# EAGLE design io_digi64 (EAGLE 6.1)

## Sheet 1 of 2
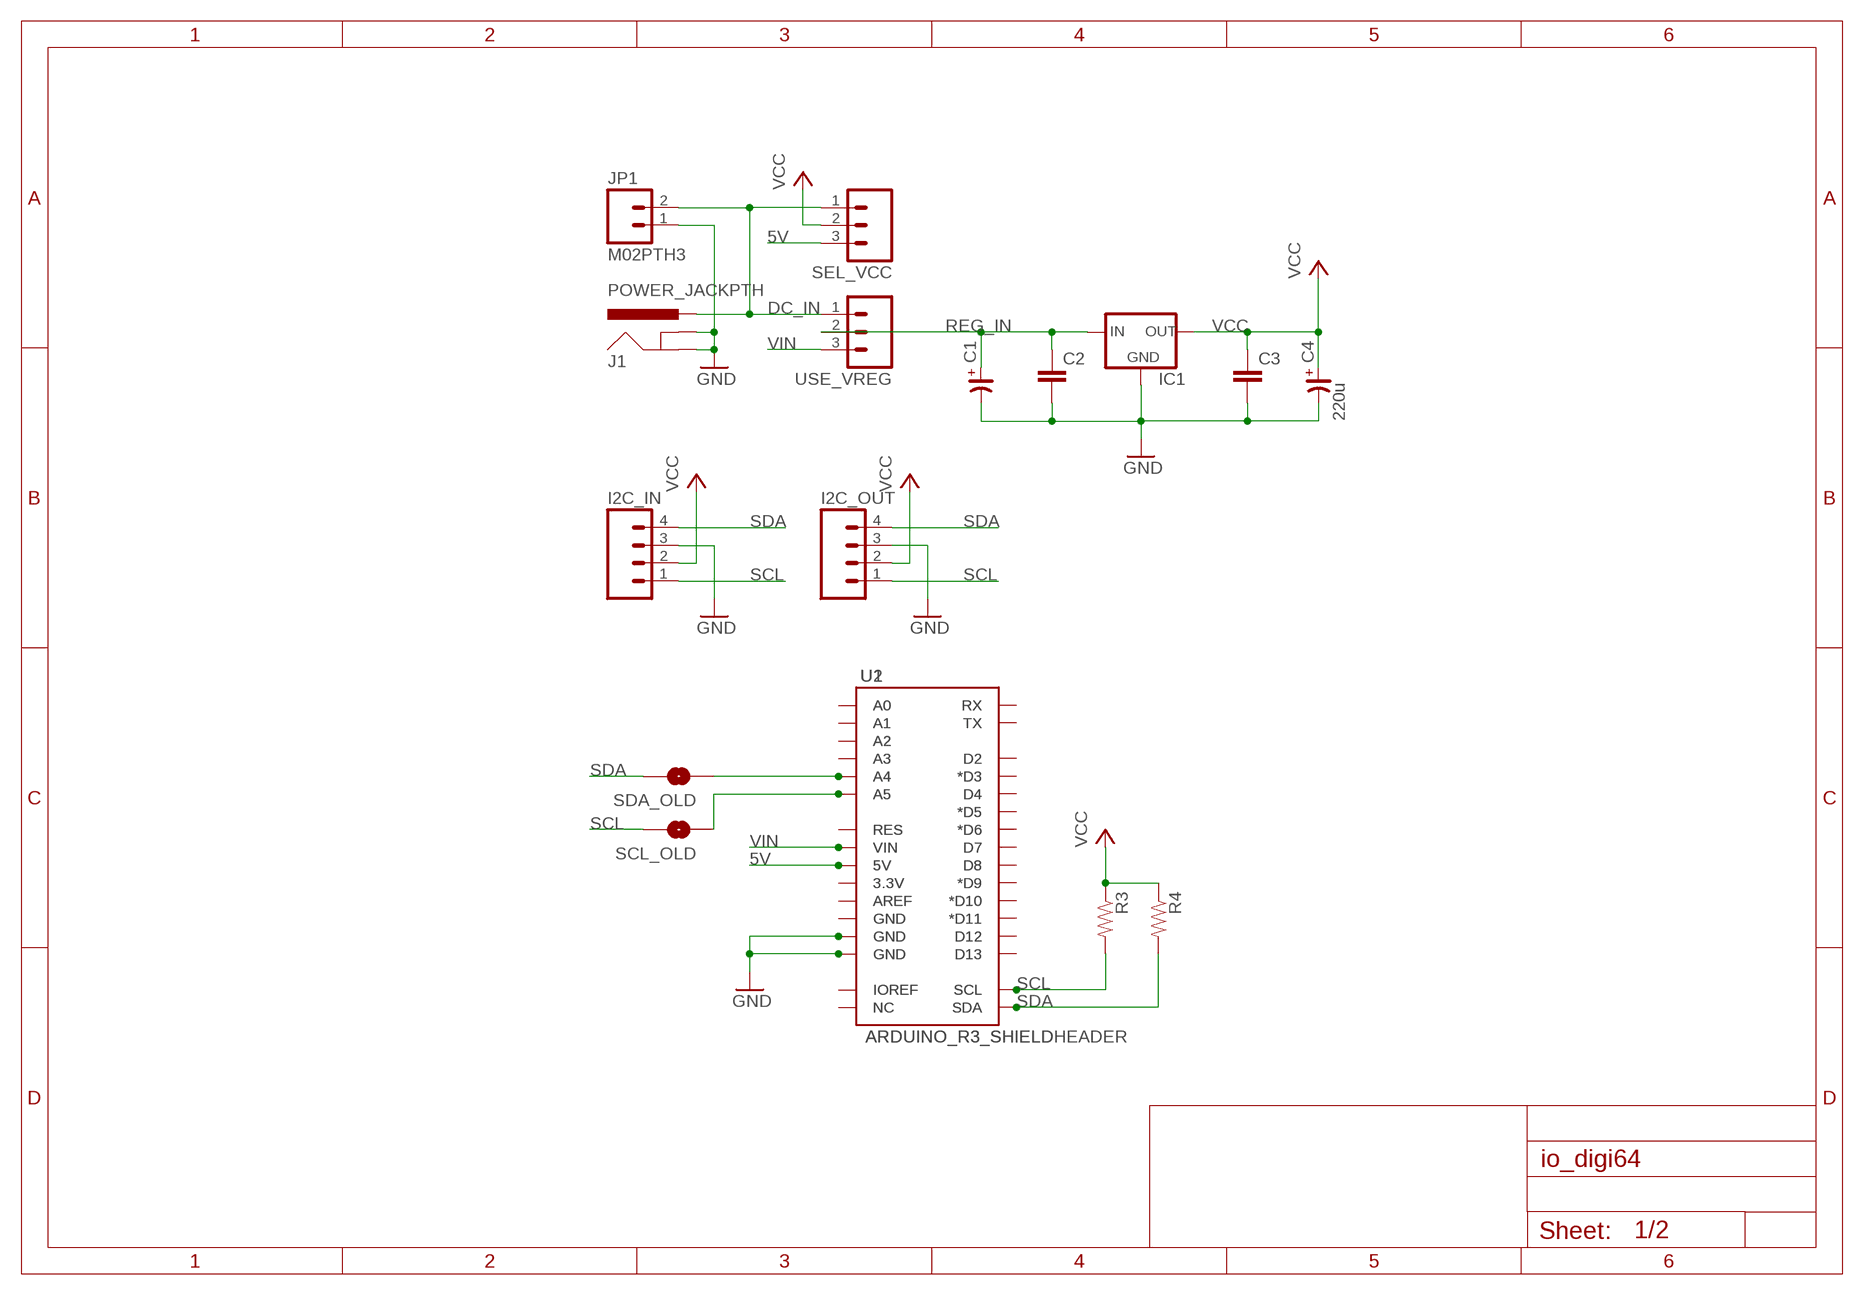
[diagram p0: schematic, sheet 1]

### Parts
C1  CP_E-025X065  [CE-025X065]
C2  CAPPTH1  [CAP-PTH-5MM]
C3  CAPPTH1  [CAP-PTH-5MM]
C4  220u  CP_E-035X080  [CE-035X080]
I2C_IN  M04PTH  [1X04]
I2C_OUT  M04PTH  [1X04]
IC1  V_REG_78XXSINK  [TO220-IGO]
J1  POWER_JACKPTH  [POWER_JACK_PTH]
JP1  M02PTH3  [1X02_LONGPADS]
R3  RESISTORPTH-1/6W  [1/6W-RES]
R4  RESISTORPTH-1/6W  [1/6W-RES]
SCL_OLD  SOLDERJUMPERNO  [SJ_2S-NO]
SDA_OLD  SOLDERJUMPERNO  [SJ_2S-NO]
SEL_VCC  M03PTH  [1X03]
U1  ARDUINO_R3_SHIELD  [ARDUINOR3_NOHOLE_NOLABELS]
U2  ARDUINO_R3_SHIELDHEADER  [ARDUINOR3_NODOC]
USE_VREG  M03PTH  [1X03]

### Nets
5V: SEL_VCC.3 U1.5V U2.5V
DC_IN: J1.PWR JP1.2 SEL_VCC.1 USE_VREG.1
GND [power]: C1.- C2.2 C3.2 C4.- I2C_IN.3 I2C_OUT.3 IC1.GND J1.GND J1.GNDBREAK JP1.1 U1.GND@0(GND) U1.GND@1(GND) U2.GND@0(GND) U2.GND@1(GND) ; also sheet 2
N$57: SDA_OLD.1 U1.A4 U2.A4
N$58: SCL_OLD.1 U1.A5 U2.A5
N$59: U1.NC U2.NC
N$60: U1.RX U2.RX
N$61: U1.TX U2.TX
N$62: U1.D2 U2.D2
N$63: U1.D3(*D3) U2.D3(*D3)
N$64: U1.D4 U2.D4
N$65: U1.D5(*D5) U2.D5(*D5)
N$66: U1.D6(*D6) U2.D6(*D6)
N$67: U1.D7 U2.D7
N$68: U1.D8 U2.D8
N$69: U1.D9(*D9) U2.D9(*D9)
N$70: U1.D10(*D10) U2.D10(*D10)
N$71: U1.D11(*D11) U2.D11(*D11)
N$72: U1.D12 U2.D12
N$73: U1.D13 U2.D13
N$74: U1.A0 U2.A0
N$75: U1.A1 U2.A1
N$76: U1.A2 U2.A2
N$77: U1.A3 U2.A3
N$79: U1.RES U2.RES
N$81: U1.AREF U2.AREF
N$82: U1.GND@2(GND) U2.GND@2(GND)
N$83: U1.3.3V U2.3.3V
N$84: U1.IOREF U2.IOREF
REG_IN: C1.+ C2.1 IC1.IN USE_VREG.2
SCL: I2C_IN.1 I2C_OUT.1 R3.2 SCL_OLD.2 U1.SCL U2.SCL ; also sheet 2
SDA: I2C_IN.4 I2C_OUT.4 R4.2 SDA_OLD.2 U1.SDA U2.SDA ; also sheet 2
VCC [power]: C3.1 C4.+ I2C_IN.2 I2C_OUT.2 IC1.OUT R3.1 R4.1 SEL_VCC.2 ; also sheet 2
VIN [power]: U1.VIN U2.VIN USE_VREG.3

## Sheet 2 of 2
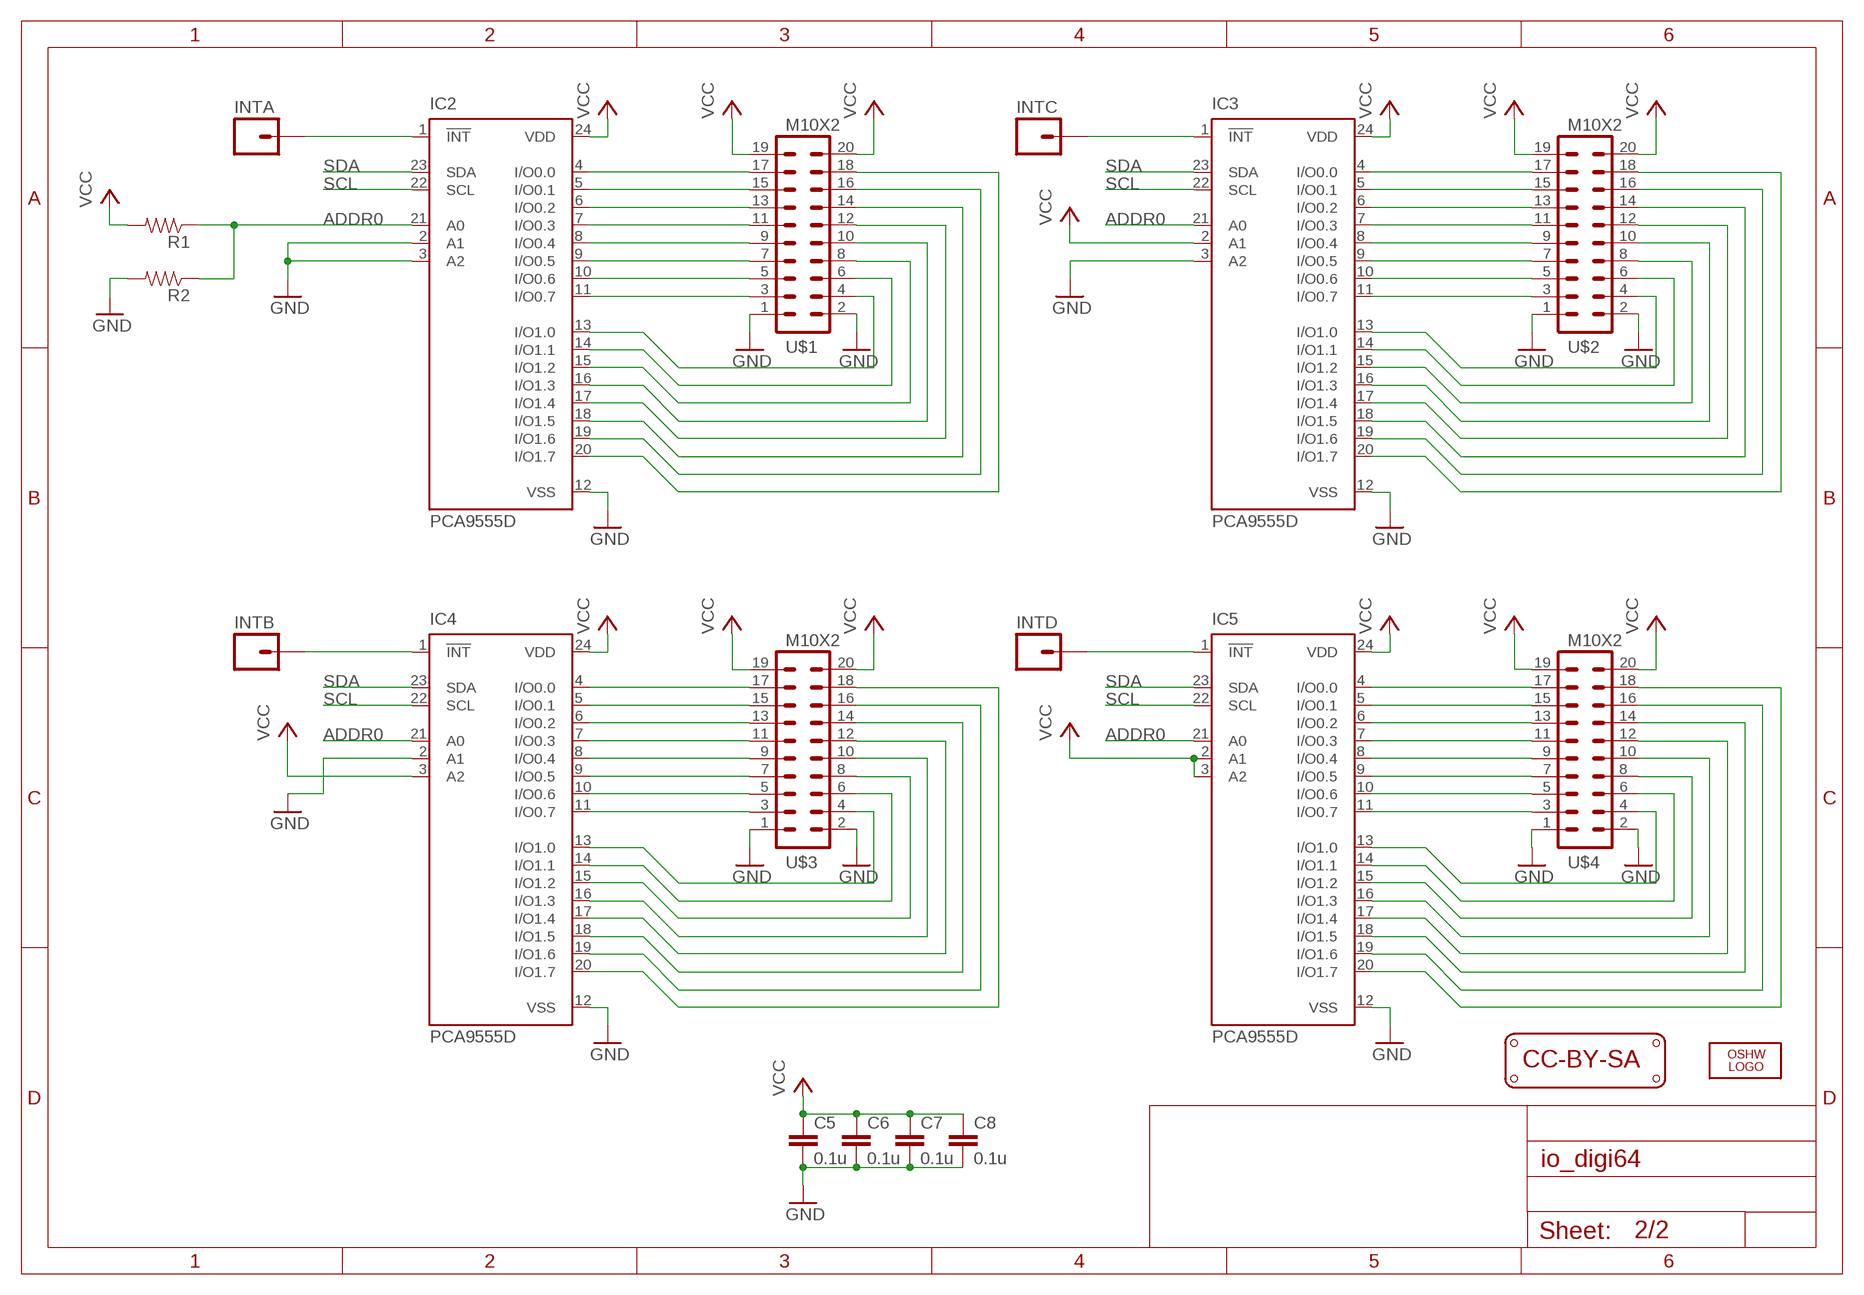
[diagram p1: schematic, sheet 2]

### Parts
C5  0.1u  CAP0805  [0805]
C6  0.1u  CAP0805  [0805]
C7  0.1u  CAP0805  [0805]
C8  0.1u  CAP0805  [0805]
IC2  PCA9555D  [SO24]
IC3  PCA9555D  [SO24]
IC4  PCA9555D  [SO24]
IC5  PCA9555D  [SO24]
INTA  M01PTH  [1X01]
INTB  M01PTH  [1X01]
INTC  M01PTH  [1X01]
INTD  M01PTH  [1X01]
LOGO1  LOGO_CC-BY-SA  [CC-BY-SA]
LOGO2  OSHW_LOGO_FILLX0200-NT  [OSHW_FILLX200_NOTEXT]
R1  RESISTORPTH-1/6W  [1/6W-RES]
R2  RESISTORPTH-1/6W  [1/6W-RES]
U$1  M10X2  [2X10]
U$2  M10X2  [2X10]
U$3  M10X2  [2X10]
U$4  M10X2  [2X10]

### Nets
ADDR0: IC2.21(A0) IC3.21(A0) IC4.21(A0) IC5.21(A0) R1.1 R2.1
GND [power]: C5.2 C6.2 C7.2 C8.2 IC2.2(A1) IC2.3(A2) IC2.12(VSS) IC3.3(A2) IC3.12(VSS) IC4.2(A1) IC4.12(VSS) IC5.12(VSS) R2.2 U$1.1 U$1.2 U$2.1 U$2.2 U$3.1 U$3.2 U$4.1 U$4.2 ; also sheet 1
N$1: IC4.13(I/O1.0) U$3.4
N$2: IC4.14(I/O1.1) U$3.6
N$3: IC4.15(I/O1.2) U$3.8
N$4: IC4.16(I/O1.3) U$3.10
N$5: IC4.17(I/O1.4) U$3.12
N$6: IC4.18(I/O1.5) U$3.14
N$7: IC4.19(I/O1.6) U$3.16
N$8: IC4.20(I/O1.7) U$3.18
N$9: IC3.11(I/O0.7) U$2.3
N$10: IC3.10(I/O0.6) U$2.5
N$11: IC3.9(I/O0.5) U$2.7
N$12: IC3.8(I/O0.4) U$2.9
N$13: IC3.7(I/O0.3) U$2.11
N$14: IC3.6(I/O0.2) U$2.13
N$15: IC3.5(I/O0.1) U$2.15
N$16: IC3.4(I/O0.0) U$2.17
N$17: IC3.13(I/O1.0) U$2.4
N$18: IC3.14(I/O1.1) U$2.6
N$19: IC3.15(I/O1.2) U$2.8
N$20: IC3.16(I/O1.3) U$2.10
N$21: IC3.17(I/O1.4) U$2.12
N$22: IC3.18(I/O1.5) U$2.14
N$23: IC3.19(I/O1.6) U$2.16
N$24: IC3.20(I/O1.7) U$2.18
N$25: IC5.11(I/O0.7) U$4.3
N$26: IC5.10(I/O0.6) U$4.5
N$27: IC5.9(I/O0.5) U$4.7
N$28: IC5.8(I/O0.4) U$4.9
N$29: IC5.7(I/O0.3) U$4.11
N$30: IC5.6(I/O0.2) U$4.13
N$31: IC5.5(I/O0.1) U$4.15
N$32: IC5.4(I/O0.0) U$4.17
N$33: IC5.13(I/O1.0) U$4.4
N$34: IC5.14(I/O1.1) U$4.6
N$35: IC5.15(I/O1.2) U$4.8
N$36: IC5.16(I/O1.3) U$4.10
N$37: IC5.17(I/O1.4) U$4.12
N$38: IC5.18(I/O1.5) U$4.14
N$39: IC5.19(I/O1.6) U$4.16
N$40: IC5.20(I/O1.7) U$4.18
N$41: IC2.11(I/O0.7) U$1.3
N$42: IC2.10(I/O0.6) U$1.5
N$43: IC2.9(I/O0.5) U$1.7
N$44: IC2.8(I/O0.4) U$1.9
N$45: IC2.7(I/O0.3) U$1.11
N$46: IC2.6(I/O0.2) U$1.13
N$47: IC2.5(I/O0.1) U$1.15
N$48: IC2.4(I/O0.0) U$1.17
N$49: IC2.13(I/O1.0) U$1.4
N$50: IC2.14(I/O1.1) U$1.6
N$51: IC2.15(I/O1.2) U$1.8
N$52: IC2.16(I/O1.3) U$1.10
N$53: IC2.17(I/O1.4) U$1.12
N$54: IC2.18(I/O1.5) U$1.14
N$55: IC2.19(I/O1.6) U$1.16
N$56: IC2.20(I/O1.7) U$1.18
N$80: IC2.1(!INT) INTA.1
N$85: IC4.1(!INT) INTB.1
N$86: IC3.1(!INT) INTC.1
N$87: IC5.1(!INT) INTD.1
N$113: IC4.11(I/O0.7) U$3.3
N$114: IC4.10(I/O0.6) U$3.5
N$115: IC4.9(I/O0.5) U$3.7
N$116: IC4.8(I/O0.4) U$3.9
N$117: IC4.7(I/O0.3) U$3.11
N$118: IC4.6(I/O0.2) U$3.13
N$119: IC4.5(I/O0.1) U$3.15
N$120: IC4.4(I/O0.0) U$3.17
SCL: IC2.22(SCL) IC3.22(SCL) IC4.22(SCL) IC5.22(SCL) ; also sheet 1
SDA: IC2.23(SDA) IC3.23(SDA) IC4.23(SDA) IC5.23(SDA) ; also sheet 1
VCC [power]: C5.1 C6.1 C7.1 C8.1 IC2.24(VDD) IC3.2(A1) IC3.24(VDD) IC4.3(A2) IC4.24(VDD) IC5.2(A1) IC5.3(A2) IC5.24(VDD) R1.2 U$1.19 U$1.20 U$2.19 U$2.20 U$3.19 U$3.20 U$4.19 U$4.20 ; also sheet 1

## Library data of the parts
C1 C4 = rc-master:CP_: POLARIZED CAP
C2 C3 C5-C8 = general:CAP: Capacitor
I2C_IN I2C_OUT = SparkFun-Connectors:M04: Header 4 Standard 4-pin 0.1" header. Use with straight break away headers (SKU : PRT-00116), right angle break away headers (PRT-00553), swiss pins (PRT-00743), machine pins (PRT-00117), and female headers (PRT-00115). Molex polarized connector foot print use with SKU : PRT-08231 with associated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
IC1 = SparkFun-PowerIC:V_REG_78XX: Voltage Regulator Standard 7805 5V regulator. IGO (Input Ground Output). Spark Fun Electronics SKU : COM-00107
IC2-IC5 = micro-philips:PCA9555: 16-bit I2C and SMBus I/O port with interrupt Source: PCA9555_5.pdf; MPN: PCA9555DW; OC_FARNELL: 1408295; OC_NEWARK: 63K6067
INTA INTB INTC INTD = SparkFun-Connectors:M01: Header 1
J1 = SparkFun-Connectors:POWER_JACK: Power Jack This is the standard 5.5mm barrel jack for power. The PTH is the most common, proven, reliable, footprint. The Slot footprint only works if the mill layer is transmitted to the PCB fab house so be warned. Spark Fun Electronics SKU : PRT-00119 SMT: CONN-08106 Mating wall wart : TOL-00298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
JP1 = SparkFun-Connectors:M02: Standard 2-pin 0.1" header. Use with
LOGO1 = dp_devices:LOGO_CC-BY-SA
LOGO2 = ohw-logo:OSHW_LOGO_FILL
R1-R4 = general:RESISTOR: Resistor
SCL_OLD SDA_OLD = SparkFun-Passives:SOLDERJUMPER: Solder Jumper
SEL_VCC USE_VREG = SparkFun-Connectors:M03: Header 3 Standard 3-pin 0.1" header. Use with straight break away headers (SKU : PRT-00116), right angle break away headers (PRT-00553), swiss pins (PRT-00743), machine pins (PRT-00117), and female headers (PRT-00115). Molex polarized connector foot print use with SKU : PRT-08232 with associated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
U1 = arduino_shield:ARDUINO_R3_SHIELD; U: ArduinoR3
U2 = arduino_shield:ARDUINO_R3_SHIELD
U$1-U$4 = SparkFun-Connectors:M10X2: This was SPECIALLY designed to be used with our Graphic LCD Backpack. Be sure you want to use this! It is not only staggered on each line of header holes, but IT IS ALSO offset of the center point of the top and bottom lines by 5 mil. This causes the headers to lock into place on the "standard"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

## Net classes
1 power: width 0.406 mm, clearance 0.203 mm

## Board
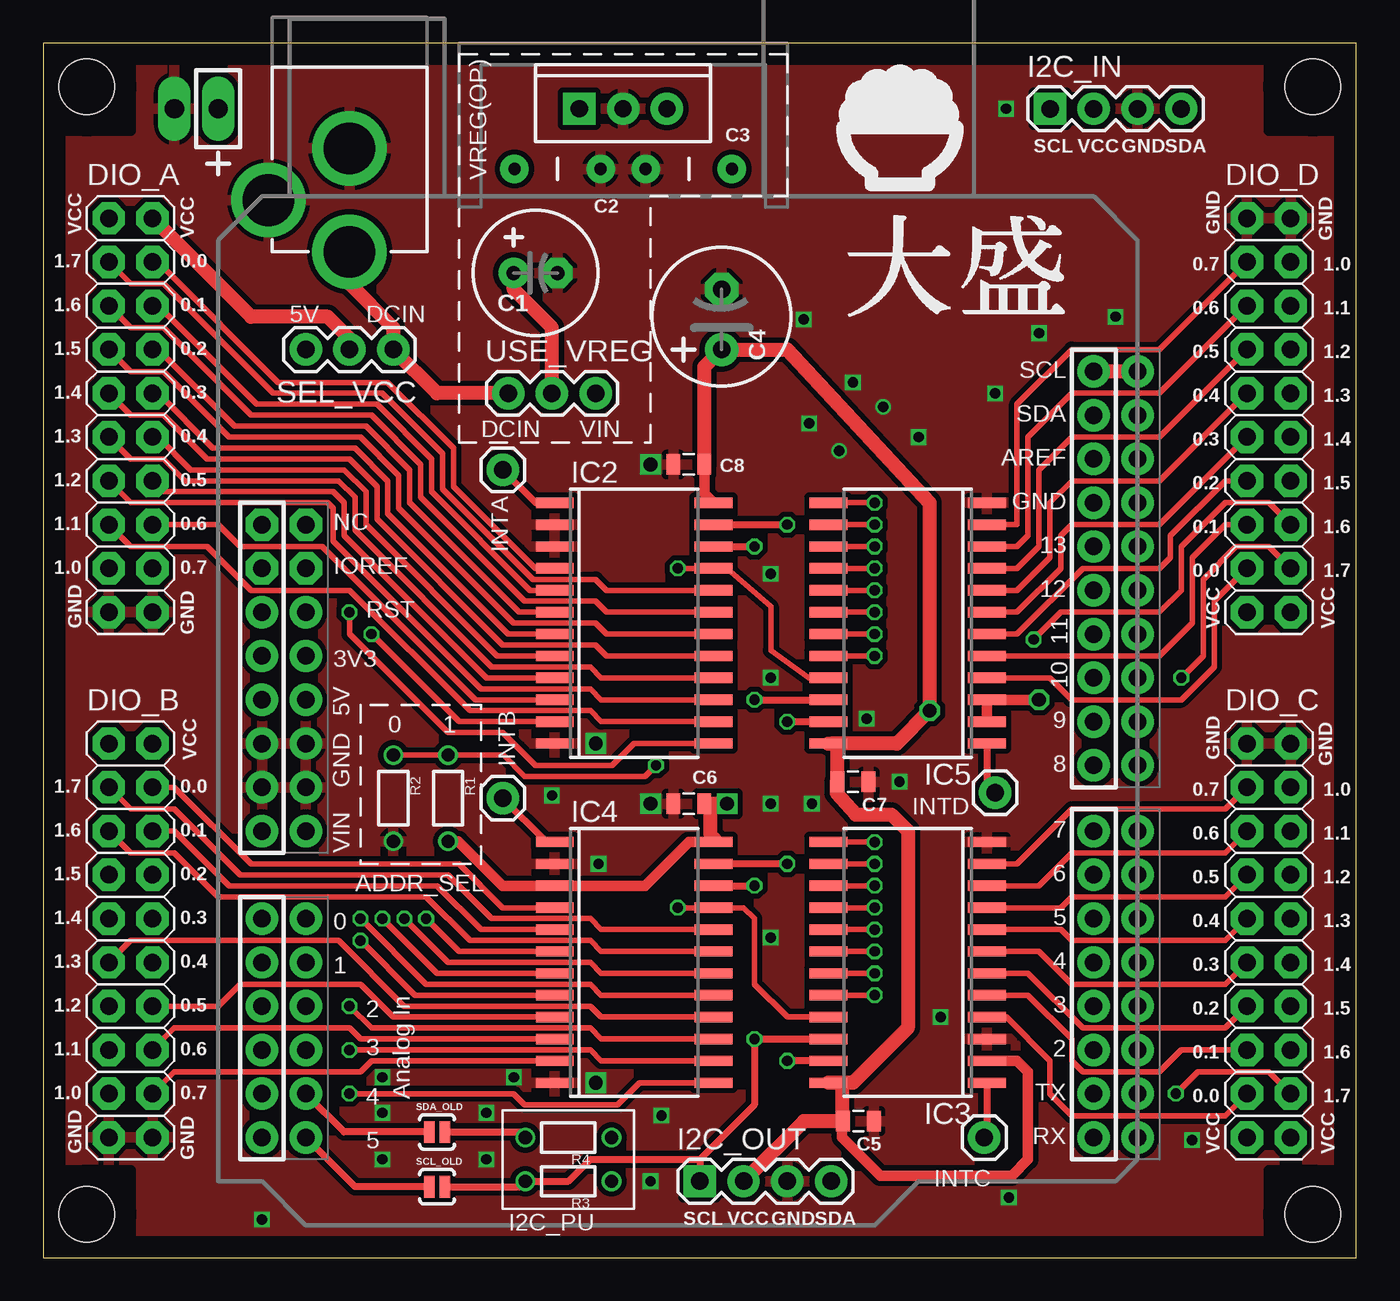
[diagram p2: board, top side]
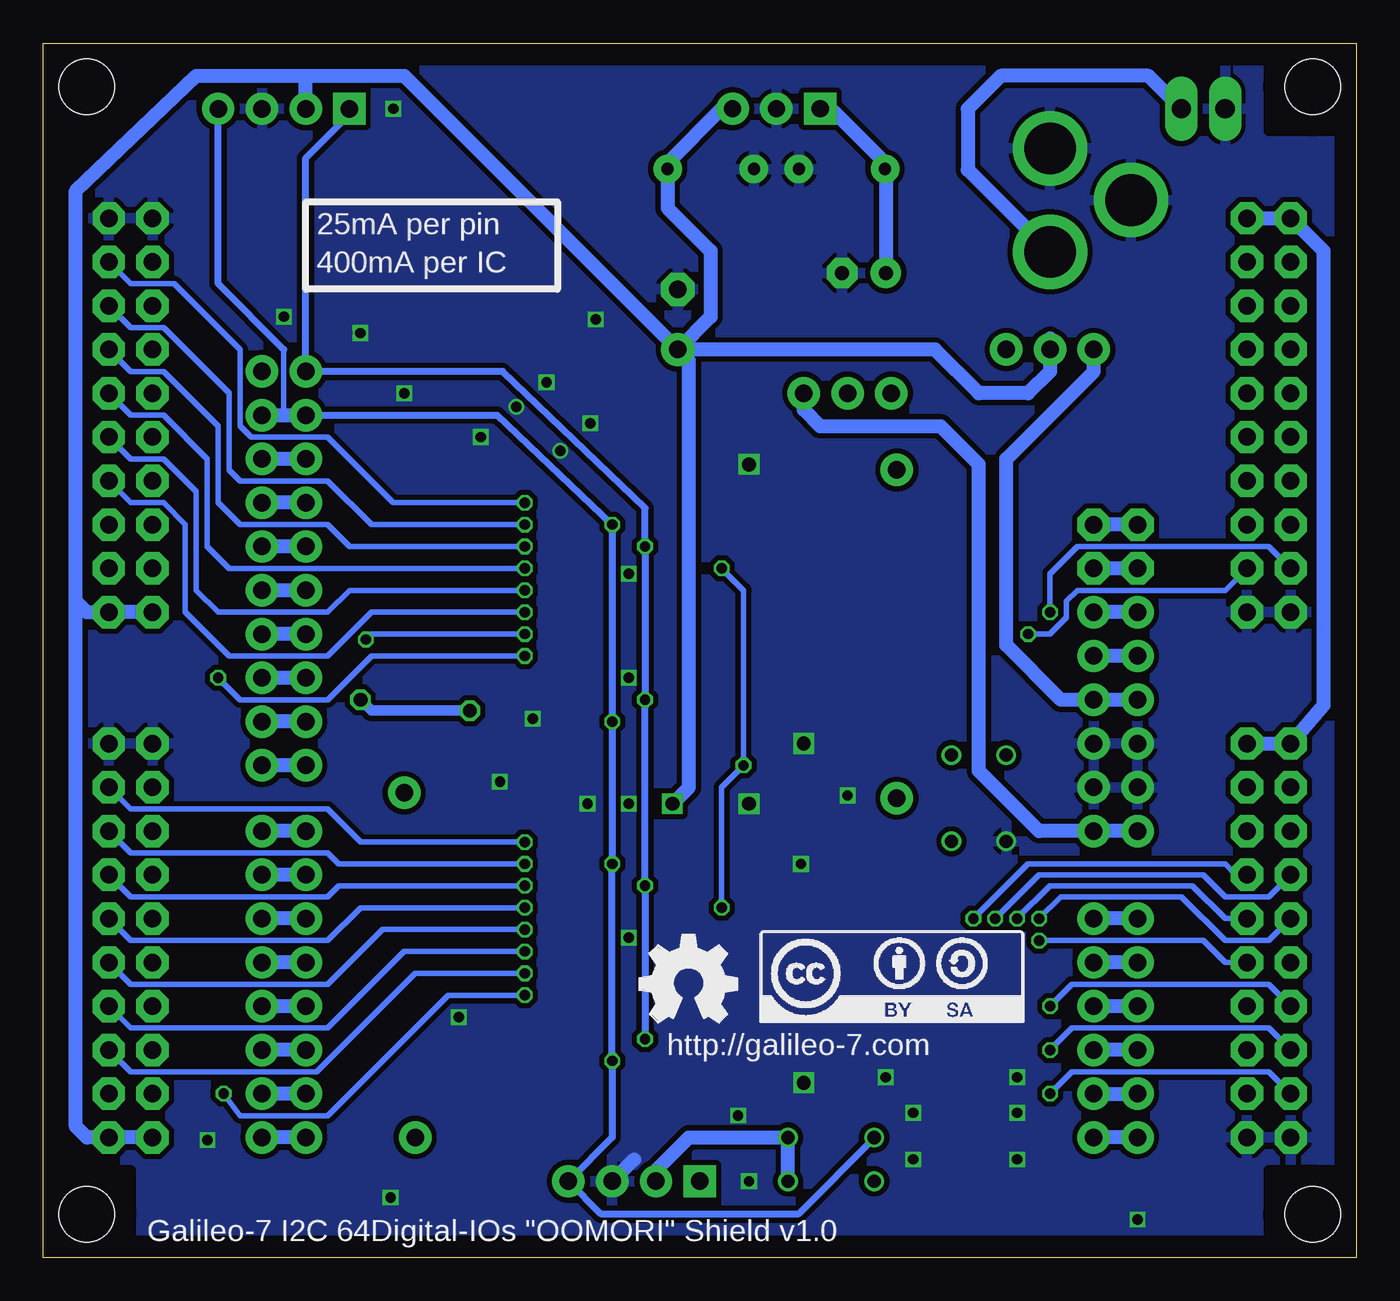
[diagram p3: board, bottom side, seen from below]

Size 76.2 x 70.48 mm. Coordinates in mm from the lower left corner, seen from the top.
Outline: 0,0 76.2,0 76.2,70.48 0,70.48 0,0
Copper layers (1*2*15*16): Top 0.035mm / dielectric 0.2mm / Route2 0.0175mm / dielectric 1.1mm / Route15 0.0175mm / dielectric 0.2mm / Bottom 0.035mm
Design rules: minimum track width 6mil, minimum drill 12mil, track to track 6mil, track to pad 6mil, pad to pad 6mil, via to via 6mil, smd to smd 0mil, copper to edge 50mil, drill to drill 10mil, minimum pad ring 6mil, minimum via ring 6mil, stop-mask expansion 2mil, vias tented up to drill 25mil, thermal gap 10mil
Holes 3.2 mm at 2.54,67.94 73.66,67.94 2.54,2.54 73.66,2.54
tRestrict: area 0,0 to 5.1,5.1; area 71.1,0 to 76.2,5.1; area 71.1,65.4 to 76.2,70.5; area 0,65.4 to 5.1,70.5
bRestrict: area 0,0 to 5.1,5.1; area 71.1,0 to 76.2,5.1; area 71.1,65.4 to 76.2,70.5; area 0,65.4 to 5.1,70.5

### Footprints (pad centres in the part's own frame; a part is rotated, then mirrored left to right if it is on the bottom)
CE-025X065 = drill 0.813 pad 1.778: + -1.27,0 | drill 0.813 pad 1.778 octagon: - 1.27,0
CAP-PTH-5MM = drill 0.7 pad 1.651: 1 -2.5,0; 2 2.5,0
CE-035X080 = drill 1.016 pad 1.93: + -1.905,0 | drill 1.016 pad 1.93 octagon: - 1.587,0
0805 = smd 0.8 x 1.2: 1 -0.9,0; 2 0.9,0
1X04 = drill 1.016 pad 1.88 square: 1 0,0 | drill 1.016 pad 1.88: 2 2.54,0; 3 5.08,0; 4 7.62,0
TO220-IGO = drill 1 pad 1.88: GND 0,0; OUT 2.54,0 | drill 1 pad 1.88 square: IN -2.54,0
SO24 = smd 0.6 x 2.2: 1 -6.985,-4.6; 2 -5.715,-4.6; 3 -4.445,-4.6; 4 -3.175,-4.6; 5 -1.905,-4.6; 6 -0.635,-4.6; 7 0.635,-4.6; 8 1.905,-4.6; 9 3.175,-4.6; 10 4.445,-4.6; 11 5.715,-4.6; 12 6.985,-4.6; 13 6.985,4.6; 14 5.715,4.6; 15 4.445,4.6; 16 3.175,4.6; 17 1.905,4.6; 18 0.635,4.6; 19 -0.635,4.6; 20 -1.905,4.6; 21 -3.175,4.6; 22 -4.445,4.6; 23 -5.715,4.6; 24 -6.985,4.6
1X01 = drill 1.016 pad 1.88: 1 0,0
POWER_JACK_PTH = drill 2.997 pad 4.318: GND 0,7.7; GNDBREAK 4.7,10.7; PWR 0,13.7
1X02_LONGPADS = drill 1.118 pad 1.88 long: 1 0,0; 2 2.54,0
1/6W-RES = drill 0.762: 1 -2.5,0; 2 2.5,0
SJ_2S-NO = smd 0.635 x 1.27: 1 -0.45,0; 2 0.45,0
1X03 = drill 1.016 pad 1.88: 1 0,0; 2 2.54,0; 3 5.08,0
ARDUINOR3_NOHOLE_NOLABELS = drill 1.016 pad 1.88: 3.3V 50.8,26.67; 5V 50.8,29.21; A0 50.8,41.91; A1 50.8,44.45; A2 50.8,46.99; A3 50.8,49.53; A4 50.8,52.07; A5 50.8,54.61; AREF 2.54,15.24; D2 2.54,49.53; D3 2.54,46.99; D4 2.54,44.45; D5 2.54,41.91; D6 2.54,39.37; D7 2.54,36.83; D8 2.54,33.02; D9 2.54,30.48; D10 2.54,27.94; D11 2.54,25.4; D12 2.54,22.86; D13 2.54,20.32; GND@0 50.8,31.75; GND@1 50.8,34.29; GND@2 2.54,17.78; RES 50.8,24.13; RX 2.54,54.61; SCL 2.54,10.16; SDA 2.54,12.7; TX 2.54,52.07; VIN 50.8,36.83 | drill 1.016 pad 1.88 octagon: IOREF 50.8,21.59; NC 50.8,19.05
ARDUINOR3_NODOC = drill 1.016 pad 1.88: 3.3V 50.8,26.67; 5V 50.8,29.21; A0 50.8,41.91; A1 50.8,44.45; A2 50.8,46.99; A3 50.8,49.53; A4 50.8,52.07; A5 50.8,54.61; AREF 2.54,15.24; D2 2.54,49.53; D3 2.54,46.99; D4 2.54,44.45; D5 2.54,41.91; D6 2.54,39.37; D7 2.54,36.83; D8 2.54,33.02; D9 2.54,30.48; D10 2.54,27.94; D11 2.54,25.4; D12 2.54,22.86; D13 2.54,20.32; GND@0 50.8,31.75; GND@1 50.8,34.29; GND@2 2.54,17.78; RES 50.8,24.13; RX 2.54,54.61; SCL 2.54,10.16; SDA 2.54,12.7; TX 2.54,52.07; VIN 50.8,36.83 | drill 1.016 pad 1.88 octagon: IOREF 50.8,21.59; NC 50.8,19.05
2X10 = drill 1.016 pad 1.88 octagon: 1 -11.43,-1.27; 2 -11.43,1.27; 3 -8.89,-1.27; 4 -8.89,1.27; 5 -6.35,-1.27; 6 -6.35,1.27; 7 -3.81,-1.27; 8 -3.81,1.27; 9 -1.27,-1.27; 10 -1.27,1.27; 11 1.27,-1.27; 12 1.27,1.27; 13 3.81,-1.27; 14 3.81,1.27; 15 6.35,-1.27; 16 6.35,1.27; 17 8.89,-1.27; 18 8.89,1.27; 19 11.43,-1.27; 20 11.43,1.27

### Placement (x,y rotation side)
C1  28.57,57.15 0 top
C2  29.84,63.18 0 top
C3  37.47,63.18 180 top
C4  39.37,54.61 90 top
C5  47.31,7.94 0 top
C6  37.47,26.35 180 top
C7  46.99,27.62 0 top
C8  37.47,46.04 180 top
I2C_IN  58.42,66.67 0 top
I2C_OUT  38.1,4.45 0 top
IC1  33.66,66.67 0 top
IC2  34.29,36.83 270 top
IC3  50.16,17.14 90 top
IC4  34.29,17.14 270 top
IC5  50.16,36.83 90 top
INTA  26.67,45.72 0 top
INTB  26.67,26.67 0 top
INTC  54.61,6.99 0 top
INTD  55.24,26.99 0 top
J1  17.78,72.07 180 top
JP1  7.62,66.67 0 top
LOGO1  34.61,13.65 0 bottom
LOGO2  41.59,13.65 0 bottom
R1  23.5,26.67 270 top
R2  20.32,26.67 270 top
R3  30.48,4.45 180 top
R4  30.48,6.99 180 top
SCL_OLD  22.86,4.13 0 top
SDA_OLD  22.86,7.3 0 top
SEL_VCC  20.32,52.7 180 top
U1  63.5,61.59 180 top
U2  66.04,61.59 180 top
U$1  5.08,48.9 90 top
U$2  71.12,18.41 270 top
U$3  5.08,18.41 90 top
U$4  71.12,48.9 270 top
U$5  [OMORI_LOGO]  46.04,61.91 0 top
U$6  [OMORI_LOGO2]  46.67,54.61 0 top
USE_VREG  26.99,50.16 0 top

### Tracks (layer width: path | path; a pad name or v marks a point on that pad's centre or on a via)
5V
  Bottom 0.813: SEL_VCC.3 15.24,51.44 20.32,46.35 20.32,35.56 17.14,32.38 U2.5V U1.5V
ADDR0  (via drill 0.6)
  Top 0.305: 45.72,33.66 IC5.21 44.45,33.66 42.23,35.24 42.23,37.78 39.69,40.01 IC2.21 v36.83,40.01 | IC3.21 43.18,13.97 41.27,15.88 41.27,19.68 40.64,20.32 IC4.21 v36.83,20.32 | R2.1 R1.1 26.71,29.17 27.94,27.94 34.92,27.94 v35.56,28.57
  Bottom 0.305: v36.83,40.01 35.56,38.73 v35.56,28.57 36.83,27.3 v36.83,20.32
DC_IN
  Top 0.813: USE_VREG.1 22.86,50.16 SEL_VCC.1 20.32,53.98 17.78,56.52 J1.PWR
  Bottom 0.813: JP1.2 12.06,68.58 20.64,68.58 22.54,66.67 22.54,63.13 J1.PWR
GND  (via drill 0.6, 0.8)
  Top 0.406: IC2.3 30.16,41.27
  Bottom 0.813: I2C_OUT.3 41.91,5.71
  other vias: 32.07,29.84 32.07,10.16 35.24,46.04 35.24,26.35 57.78,53.66 55.88,66.67 46.99,50.8 55.24,50.16 44.45,48.42 62.23,54.61 42.23,39.69 42.23,33.66 42.23,26.35 42.23,18.57 46.2,46.83 48.74,49.37 29.53,26.83 35.88,8.26 27.3,10.48 19.68,10.48 44.13,54.45 47.78,31.27 56.04,3.49 32.23,22.86 50.8,47.62 44.61,26.35 49.69,27.62 52.07,13.97 12.7,2.22 66.67,6.83 19.68,8.41 25.72,8.41 25.72,5.71 19.68,5.71 35.24,4.45
  pour Top (isolate 0.305): 0,70.48 76.2,70.48 76.2,0 0,0
  pour Bottom (isolate 0.305): 0,70.48 0,5.08 0,0 76.2,0 76.2,70.48
N$1  (via drill 0.6)
  Top 0.305: IC4.13 34.61,10.16 33.34,8.89 27.94,8.89 27.3,9.53 v17.78,9.53
  Bottom 0.305: U$3.4 5.08,10.79 16.51,10.79 v17.78,9.53
N$2  (via drill 0.6)
  Top 0.305: v17.78,12.06 31.75,12.06 32.38,11.43 IC4.14
  Bottom 0.305: U$3.6 5.08,13.34 16.51,13.34 v17.78,12.06
N$3  (via drill 0.6)
  Top 0.305: v17.78,14.61 19.05,13.34 31.75,13.34 32.38,12.7 IC4.15
  Bottom 0.305: U$3.8 5.08,15.88 16.51,15.88 v17.78,14.61
N$4
  Top 0.305: IC4.16 32.38,13.97 31.75,14.61 20.95,14.61 17.14,18.41 5.08,18.41 U$3.10
N$5  (via drill 0.6)
  Top 0.305: v18.41,19.68 22.23,15.88 31.75,15.88 32.38,15.24 IC4.17
  Bottom 0.305: U$3.12 5.08,18.41 7.62,18.41 10.16,20.95 17.14,20.95 v18.41,19.68
N$6  (via drill 0.6)
  Top 0.305: v20.95,19.68 23.5,17.14 31.75,17.14 32.38,16.51 IC4.18 39.37,16.51
  Bottom 0.305: U$3.14 5.08,20.95 7.62,20.95 8.89,22.23 18.41,22.23 v20.95,19.68
N$7
  Top 0.305: IC4.19 32.38,17.78 31.75,18.41 24.77,18.41 22.23,20.95 10.16,20.95 7.62,23.5 5.08,23.5 U$3.16
N$8
  Top 0.305: U$3.18 5.08,26.04 7.62,26.04 11.43,22.23 23.5,22.23 26.04,19.68 31.75,19.68 32.38,19.05 IC4.20
N$9
  Top 0.305: IC3.11 56.52,22.86 59.69,26.04 68.58,26.04 U$2.3
N$10
  Top 0.305: IC3.10 57.78,21.59 59.69,23.5 68.58,23.5 U$2.5
N$11
  Top 0.305: IC3.9 59.05,20.32 59.69,20.95 68.58,20.95 U$2.7
N$12
  Top 0.305: IC3.8 59.05,19.05 59.69,18.41 68.58,18.41 U$2.9
N$13
  Top 0.305: IC3.7 57.78,17.78 59.69,15.88 68.58,15.88 U$2.11
N$14
  Top 0.305: U$2.13 68.58,13.34 60.33,13.34 57.15,16.51 IC3.6
N$15
  Top 0.305: IC3.5 57.15,15.24 59.69,12.7 59.69,11.43 60.33,10.79 64.77,10.79 66.04,12.06 U$2.15
N$16
  Top 0.305: IC3.4 55.88,13.97 58.42,11.43 58.42,9.53 59.69,8.26 68.58,8.26 U$2.17
N$17  (via drill 0.6)
  Top 0.305: v48.26,24.13 IC3.13
  Bottom 0.305: U$2.4 71.12,26.04 59.69,26.04 57.78,24.13 v48.26,24.13
N$18  (via drill 0.6)
  Top 0.305: IC3.14 v48.26,22.86
  Bottom 0.305: v48.26,22.86 59.05,22.86 59.69,23.5 71.12,23.5 U$2.6
N$19  (via drill 0.6)
  Top 0.305: IC3.15 v48.26,21.59
  Bottom 0.305: v48.26,21.59 59.05,21.59 59.69,20.95 71.12,20.95 U$2.8
N$20  (via drill 0.6)
  Top 0.305: IC3.16 v48.26,20.32
  Bottom 0.305: v48.26,20.32 57.78,20.32 59.69,18.41 71.12,18.41 U$2.10
N$21  (via drill 0.6)
  Top 0.305: v48.26,19.05 IC3.17
  Bottom 0.305: U$2.12 71.12,15.88 59.69,15.88 56.52,19.05 v48.26,19.05
N$22  (via drill 0.6)
  Top 0.305: IC3.18 v48.26,17.78
  Bottom 0.305: v48.26,17.78 55.24,17.78 59.69,13.34 71.12,13.34 U$2.14
N$23  (via drill 0.6)
  Top 0.305: v48.26,16.51 IC3.19
  Bottom 0.305: U$2.16 71.12,10.79 60.33,10.79 54.61,16.51 v48.26,16.51
N$24  (via drill 0.6)
  Top 0.305: IC3.20 v48.26,15.24 | U$2.18 71.12,10.79 66.99,10.79 v65.72,9.53
  Bottom 0.305: v65.72,9.53 64.77,8.26 59.69,8.26 52.7,15.24 v48.26,15.24
N$25
  Top 0.305: IC5.11 56.52,42.55 56.52,49.53 59.69,52.7 64.77,52.7 U$4.3
N$26
  Top 0.305: IC5.10 56.52,41.27 57.15,41.91 57.15,47.62 59.69,50.16 64.77,50.16 U$4.5
N$27
  Top 0.305: IC5.9 56.52,40.01 57.78,41.27 57.78,45.72 59.69,47.62 64.77,47.62 U$4.7
N$28
  Top 0.305: IC5.8 56.52,38.73 58.42,40.64 58.42,43.81 59.69,45.09 64.77,45.09 U$4.9
N$29
  Top 0.305: IC5.7 56.52,37.47 59.05,40.01 59.05,41.91 59.69,42.55 64.77,42.55 U$4.11
N$30
  Top 0.305: IC5.6 56.52,36.2 60.33,40.01 64.77,40.01 65.41,40.64 65.41,41.91 68.58,45.09 U$4.13
N$31
  Top 0.305: IC5.5 64.77,34.92 66.67,36.83 66.67,40.64 68.58,42.55 U$4.15
N$32
  Top 0.305: IC5.4 58.42,33.66 59.69,32.38 66.04,32.38 67.94,34.29 67.94,38.1 U$4.17
N$33  (via drill 0.6)
  Top 0.305: v48.26,43.81 IC5.13
  Bottom 0.305: U$4.4 71.12,56.52 68.58,56.52 64.77,52.7 64.77,48.26 64.14,47.62 59.69,47.62 55.88,43.81 v48.26,43.81
N$34  (via drill 0.6)
  Top 0.305: IC5.14 v48.26,42.55
  Bottom 0.305: v48.26,42.55 57.15,42.55 59.69,45.09 64.77,45.09 65.41,45.72 65.41,50.16 69.22,53.98 71.12,53.98 U$4.6
N$35  (via drill 0.6)
  Top 0.305: IC5.15 v48.26,41.27
  Bottom 0.305: v48.26,41.27 58.42,41.27 59.69,42.55 64.77,42.55 66.04,43.81 66.04,48.26 69.22,51.44 71.12,51.44 U$4.8
N$36  (via drill 0.6)
  Top 0.305: IC5.16 v48.26,40.01
  Bottom 0.305: v48.26,40.01 65.41,40.01 66.67,41.27 66.67,46.35 69.22,48.9 71.12,48.9 U$4.10
N$37  (via drill 0.6)
  Top 0.305: IC5.17 v48.26,38.73
  Bottom 0.305: v48.26,38.73 58.42,38.73 59.69,37.47 66.04,37.47 67.31,38.73 67.31,44.45 69.22,46.35 71.12,46.35 U$4.12
N$38  (via drill 0.6)
  Top 0.305: IC5.18 v48.26,37.47
  Bottom 0.305: v48.26,37.47 57.15,37.47 59.69,34.92 65.41,34.92 67.94,37.47 67.94,42.55 69.22,43.81 71.12,43.81 U$4.14
N$39  (via drill 0.6)
  Top 0.305: IC5.19 v48.26,36.2 | U$4.16 71.12,43.81 68.58,43.81 66.04,41.27 66.04,38.73 64.77,37.47 59.05,37.47 v57.47,35.88
  Bottom 0.305: 55.88,36.2 v48.26,36.2 57.15,36.2 v57.47,35.88
N$40  (via drill 0.6)
  Top 0.305: IC5.20 v48.26,34.92 | v66.04,33.66 67.31,34.92 67.31,39.37 69.22,41.27 71.12,41.27 U$4.18
  Bottom 0.305: v48.26,34.92 57.15,34.92 59.69,32.38 64.77,32.38 v66.04,33.66
N$41  (via drill 0.6)
  Top 0.305: IC2.11 24.13,31.11 v19.05,36.2
  Bottom 0.305: v19.05,36.2 17.78,36.2 16.83,37.15 16.83,38.1 16.19,38.73 7.62,38.73 U$1.3
N$42
  Top 0.305: IC2.10 25.08,32.38 16.19,41.27 11.43,41.27 10.16,42.55 U$1.5
N$43
  Top 0.305: IC2.9 25.72,33.66 17.46,41.91 17.46,43.81 16.83,44.45 6.99,44.45 U$1.7
N$44
  Top 0.305: IC2.8 26.35,34.92 18.73,42.55 18.73,44.45 17.46,45.72 8.57,45.72 6.67,47.62 U$1.9
N$45
  Top 0.305: IC2.7 26.99,36.2 20,43.18 20,45.09 18.1,46.99 9.84,46.99 6.67,50.16 U$1.11
N$46
  Top 0.305: IC2.6 27.62,37.47 21.27,43.81 21.27,45.72 18.73,48.26 11.11,48.26 6.67,52.7 U$1.13
N$47
  Top 0.305: 30.16,38.73 IC2.5 28.26,38.73 22.54,44.45 22.54,46.35 19.37,49.53 12.38,49.53 6.67,55.24 U$1.15
N$48
  Top 0.305: U$1.17 6.67,57.47 6.99,57.47 13.65,50.8 20,50.8 23.81,46.99 23.81,44.77 28.57,40.01 IC2.4
N$49  (via drill 0.6)
  Top 0.305: IC2.13 34.29,29.84 33.02,28.57 28.57,28.57 26.67,30.48 23.5,30.48 17.78,36.2 v17.78,37.47
  Bottom 0.305: U$1.4 5.08,41.27 16.19,41.27 17.78,39.69 v17.78,37.47
N$50
  Top 0.305: IC2.14 32.38,31.11 31.75,31.75 24.77,31.75 17.78,38.73 12.06,38.73 9.53,41.27 5.08,41.27 U$1.6
N$51
  Top 0.305: IC2.15 32.38,32.38 31.75,33.02 25.4,33.02 16.83,41.59 16.83,43.5 16.51,43.81 5.08,43.81 U$1.8
N$52
  Top 0.305: IC2.16 32.38,33.66 31.75,34.29 26.04,34.29 18.1,42.23 18.1,44.13 17.14,45.09 8.26,45.09 6.99,46.35 5.08,46.35 U$1.10
N$53
  Top 0.305: IC2.17 32.7,34.92 32.07,35.56 26.67,35.56 19.37,42.86 19.37,44.77 17.78,46.35 9.53,46.35 6.99,48.9 5.08,48.9 U$1.12
N$54
  Top 0.305: IC2.18 32.7,36.2 32.07,36.83 27.3,36.83 20.64,43.5 20.64,45.4 18.41,47.62 10.79,47.62 6.99,51.44 5.08,51.44 U$1.14
N$55
  Top 0.305: IC2.19 32.7,37.47 32.07,38.1 27.94,38.1 21.91,44.13 21.91,46.04 19.05,48.9 12.06,48.9 6.99,53.98 5.08,53.98 U$1.16
N$56
  Top 0.305: IC2.20 32.7,38.73 32.07,39.37 28.42,39.37 23.18,44.61 23.18,46.67 19.68,50.16 13.34,50.16 6.99,56.52 5.08,56.52 U$1.18
N$57
  Top 0.406: U2.A4 17.46,7.3 SDA_OLD.1
  Bottom 0.813: U2.A4 U1.A4
N$58
  Top 0.406: SCL_OLD.1 18.1,4.13 U2.A5
  Bottom 0.813: U1.A5 U2.A5
N$59
  Bottom 0.813: U1.NC U2.NC
N$60
  Bottom 0.813: U1.RX U2.RX
N$61
  Bottom 0.813: U1.TX U2.TX
N$62
  Bottom 0.813: U1.D2 U2.D2
N$63
  Bottom 0.813: U1.D3 U2.D3
N$64
  Bottom 0.813: U1.D4 U2.D4
N$65
  Bottom 0.813: U1.D5 U2.D5
N$66
  Bottom 0.813: U1.D6 U2.D6
N$67
  Bottom 0.813: U1.D7 U2.D7
N$68
  Bottom 0.813: U1.D8 U2.D8
N$69
  Bottom 0.813: U1.D9 U2.D9
N$70
  Bottom 0.813: U1.D10 U2.D10
N$71
  Bottom 0.813: U1.D11 U2.D11
N$72
  Bottom 0.813: U1.D12 U2.D12
N$73
  Bottom 0.813: U1.D13 U2.D13
N$74
  Bottom 0.813: U1.A0 U2.A0
N$75
  Bottom 0.813: U1.A1 U2.A1
N$76
  Bottom 0.813: U1.A2 U2.A2
N$77
  Bottom 0.813: U1.A3 U2.A3
N$79
  Bottom 0.813: U1.RES U2.RES
N$80
  Top 0.305: IC2.1 30.16,43.81
  Top 0.406: IC2.1 28.57,43.81 INTA.1
N$81
  Bottom 0.813: U1.AREF U2.AREF
N$82
  Bottom 0.813: U1.GND@2 U2.GND@2
N$83
  Bottom 0.813: U1.3.3V U2.3.3V
N$84
  Bottom 0.813: U1.IOREF U2.IOREF
N$85
  Top 0.406: IC4.1 29.21,24.13 INTB.1
N$86
  Top 0.406: IC3.1 54.77,7.14 INTC.1
N$87
  Top 0.406: IC5.1 54.77,27.47 INTD.1
N$113
  Top 0.305: IC4.11 19.05,11.43 18.41,10.79 7.62,10.79 U$3.3
N$114
  Top 0.305: IC4.10 18.41,12.7 17.78,13.34 7.62,13.34 U$3.5
N$115
  Top 0.305: U$3.7 10.16,14.61 11.43,15.88 18.41,15.88 20.32,13.97 IC4.9
N$116  (via drill 0.6)
  Top 0.305: IC4.8 21.59,15.24 v18.41,18.41
  Bottom 0.305: v18.41,18.41 8.89,18.41 7.62,17.14 U$3.9
N$117  (via drill 0.6)
  Top 0.305: IC4.7 22.86,16.51 v19.68,19.68
  Bottom 0.305: v19.68,19.68 17.78,21.59 9.53,21.59 7.62,19.68 U$3.11
N$118  (via drill 0.6)
  Top 0.305: v22.23,19.68 24.13,17.78 IC4.6 29.84,17.78
  Bottom 0.305: U$3.13 6.99,22.23 7.62,22.86 19.05,22.86 v22.23,19.68
N$119
  Top 0.305: IC4.5 25.4,19.05 22.86,21.59 10.79,21.59 7.62,24.77 U$3.15
N$120
  Top 0.305: U$3.17 7.62,27.3 12.06,22.86 24.13,22.86 26.67,20.32 IC4.4
REG_IN
  Top 0.813: USE_VREG.2 29.53,53.98 27.3,56.2 C1.+
  Bottom 0.813: 27.3,63.5 27.3,62.87 27.34,62.83 27.3,62.78 C1.+ | C2.1 27.34,63.46 27.3,63.5 | IC1.IN 30.48,66.67 27.3,63.5
SCL  (via drill 0.6)
  Top 0.406: IC2.22 v41.27,41.27 | v41.27,32.38 IC5.22 | IC4.22 v41.27,21.59 | IC3.22 v41.27,12.7 41.27,8.89 38.1,5.71 | 38.1,5.71 I2C_OUT.1 | 38.1,5.71 31.75,5.71 30.48,4.45 R3.2 27.66,4.13 SCL_OLD.2
  Top 0.813: U2.SCL U1.SCL
  Bottom 0.406: v41.27,12.7 v41.27,21.59 v41.27,32.38 v41.27,41.27 41.27,43.5 49.53,51.44 U1.SCL 60.96,63.82 58.42,66.36 I2C_IN.1
SDA  (via drill 0.6)
  Top 0.406: IC2.23 v43.18,42.55 | v43.18,31.11 IC5.23 | v43.18,22.86 IC4.23 | IC3.23 v43.18,11.43 | SDA_OLD.2 27.62,7.3 27.94,6.99 R4.2
  Bottom 0.305: 62.23,48.9 62.23,52.7
  Bottom 0.406: v43.18,42.55 43.18,41.27 | v43.18,42.55 v43.18,31.11 v43.18,22.86 v43.18,11.43 43.18,6.99 I2C_OUT.4 43.81,2.54 32.38,2.54 27.98,6.95 R4.2 | U1.SDA 49.85,48.9 v43.18,42.55 | 62.23,52.7 66.04,56.52 I2C_IN.4
  Bottom 0.813: U2.SDA 62.23,48.9 U1.SDA
VCC  (via drill 0.8)
  Top 0.61: C8.1 38.37,44.34 IC2.24 | 39,24.24 IC4.24 37.47,24.13 34.92,21.59 IC4.3 26.67,21.59 24.09,24.17 R1.2 | C5.1 46.41,7.67 | IC5.2 IC5.3 v57.78,32.38 | IC3.2 56.52,11.43 57.15,10.79 57.15,5.71 56.2,4.76 48.58,4.76 46.35,6.99 46.35,7.94
  Top 0.813: U$1.19 12.06,54.61 16.51,54.61 17.78,53.34 SEL_VCC.2 | C8.1 38.37,51.7 C4.+ 43.18,52.7 51.44,43.81 v51.44,31.75 49.53,29.84 45.72,29.84 | v39.69,26.35 C6.1 38.42,26.35 38.73,26.04 38.73,24.5 39,24.24 | 45.72,29.84 arc-90 46.09,29.48 C7.1 46.04,27.62 46.04,26.99 47.15,25.72 49.21,25.72 50.16,24.77 50.16,13.34 46.99,10.16 46.35,10.16 | 46.35,10.16 IC3.24 | I2C_OUT.2 44.13,7.94 46.35,7.94 C5.1 46.35,7.99 46.35,10.16 | IC5.24 45.72,29.84
  Bottom 0.61: U$2.19 U$2.20 | v57.78,32.38 57.15,31.75 v51.44,31.75
  Bottom 0.813: U$1.19 U$1.20 1.91,58.42 1.91,32.07 U$3.20 U$3.19 | C4.+ 37.47,54.61 37.47,58.42 39.97,60.92 C3.1 39.97,63.46 40.01,63.5 36.83,66.67 IC1.OUT | C4.+ 38.73,52.07 38.73,27.3 v39.69,26.35 | I2C_IN.2 60.96,68.58 | 60.96,68.58 55.24,68.58 C4.+ | I2C_OUT.2 40.64,5.08 38.73,6.99 33.02,6.99 | U$2.19 73.66,6.99 74.3,7.62 74.3,38.1 | U$4.19 U$4.20 73.66,37.47 74.3,38.1 | 74.3,38.1 74.3,61.91 67.31,68.58 60.96,68.58 | 17.78,53.34 SEL_VCC.2 17.78,51.44 19.05,50.16 21.91,50.16 24.45,52.7 C4.+ | R3.1 32.98,6.95 33.02,6.99 | R4.1 33.02,6.99
VIN
  Bottom 0.813: USE_VREG.3 32.07,49.21 31.11,48.26 24.13,48.26 21.91,46.04 21.91,28.26 18.41,24.77 U2.VIN U1.VIN

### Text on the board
tPlace: SCL | VCC | GND | SDA | VREG(OP) | DIO_A | VCC | DIO_D | GND | VCC | GND | 0.7 | 1.0 | 1.7 | 0.0 | 0.6 | 1.1 | 1.6 | 0.1 | 5V | DCIN | 0.5 | 1.2 | 1.5 | 0.2 | SCL | 1.4 | 0.3 | SDA | 0.4 | 1.3 | DCIN | VIN | 0.3 | 1.4 | 1.3 | 0.4 | AREF | 1.2 | 0.5 | 0.2 | 1.5 | GND | 0.1 | 1.6 | 1.1 | 0.6 | NC | 13 | 1.0 | 0.7 | IOREF | 0.0 | 1.7 | GND | 12 | GND | RST | 11 | VCC | VCC | 10 | 3V3 | DIO_B | 9 | DIO_C | 5V | GND | 0 | 1 | VCC | 8 | GND | 0.7 | 1.0 | 1.7 | 0.0 | GND | 7 | 0.6 | 1.1 | 1.6 | 0.1 | VIN | 6 | 0.5 | 1.2 | 1.5 | 0.2 | ADDR_SEL | 5 | 0.4 | 1.3 | 1.4 | 0.3 | 0 | 4 | 1.3 | 0.4 | 1 | 0.3 | 1.4 | 3 | 0.2 | 1.5 | 1.2 | 0.5 | 2 | 2 | 1.1 | 0.6 | 3 | 0.1 | 1.6 | TX | 0.0 | 1.7 | 1.0 | 0.7 | 4 | Analog In | GND | RX | GND | 5 | VCC | VCC | I2C_PU | SCL | VCC | GND | SDA
bPlace: 25mA per pin | 400mA per IC | http://galileo-7.com | Galileo-7 I2C 64Digital-IOs "OOMORI" Shield v1.0

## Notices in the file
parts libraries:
SparkFun-Connectors: Licensing: CC v3.0 Share-Alike You are welcome to use this library for commercial purposes.
rc-master: Copyright (C) 2007, Bob Starr
